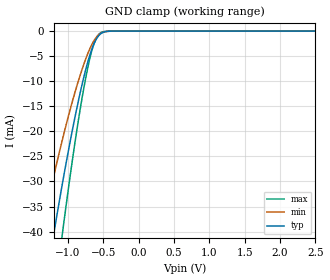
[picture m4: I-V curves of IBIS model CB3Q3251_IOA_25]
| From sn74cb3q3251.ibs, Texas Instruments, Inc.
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[Model]   CB3Q3251_IOA_25
Model_type  Terminator
| variable   typ   min   max
C_comp   2.33pF   1.81pF   2.77pF
| C_tri-state   2.33pF   1.81pF   2.77pF
[Temperature Range]   40   100   -40
| Ambient temperature   25   85   -40
[Voltage range]   2.5   2.3   2.7
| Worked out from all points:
|   GND clamp passes 1 mA (typ) near -0.57 V on its own axis
[GND Clamp]
| CB3Q3251_IOA_25
|   Voltage   I(typ)   I(min)   I(max)
-5.5V     -546.9mA   -436.2mA   -659.1mA
-1.38V    -56.54mA   -40.68mA   -75.66mA
-1.355V   -54.21mA   -38.97mA   -72.56mA
-1.195V   -40.01mA   -28.58mA   -53.44mA
-1.085V   -30.93mA   -22.02mA   -41.09mA
-1.065V   -29.35mA   -20.88mA   -38.92mA
-905mV    -17.47mA   -12.42mA   -22.63mA
-740mV    -7.209mA   -5.232mA   -8.708mA
-645mV    -2.972mA   -2.231mA   -3.063mA
-545mV    -629.6uA   -509.5uA   -405uA
-335mV    -2.907uA   -4.569uA   -281.8nA
2.5V      106.1pA    500.1pA    14.3pA
